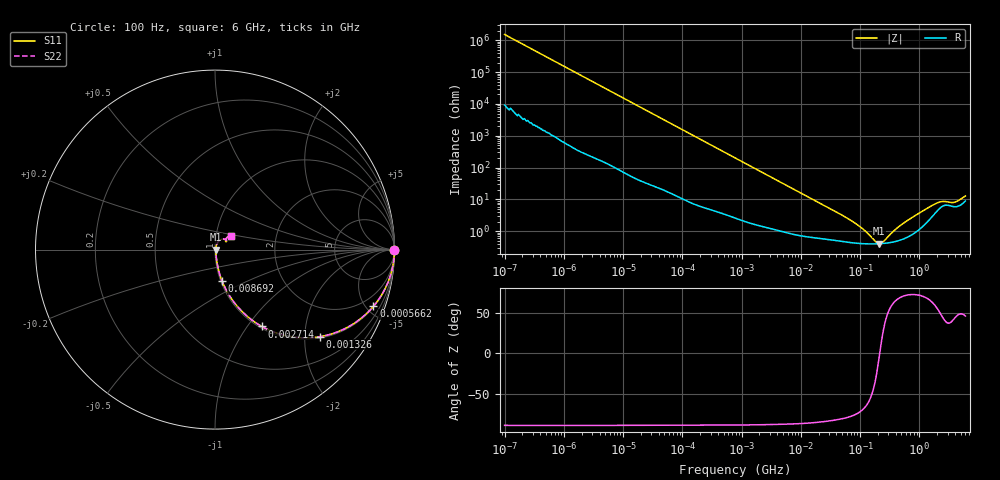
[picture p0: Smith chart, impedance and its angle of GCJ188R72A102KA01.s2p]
!Murata Part Number: GCJ188R72A102KA01
!These Parameters are Measured in Series Mode Connection
!Data Generated on Mar 13, 2026
!  o--ll--o
!Port1  Port2
!  o------o
!Operation Temp=25[degC], DC Bias Voltage=0[V]
!Freq. Start=100[Hz] Stop=6[GHz] 401[Steps]
# Hz S RI R 50
!Freq.(Hz) S11(Real) S11(Imag) S21(Real) S21(Imag) S12(Real) S12(Imag) S22(Real) S22(Imag)
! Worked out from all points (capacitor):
!   401 points, 100 Hz to 6 GHz, reference 50 ohm
!   read as one part in series: C = 1.04 nF near 109 Hz
!   lowest |Z| = 408 mohm at 208.8 MHz (marker M1)
!   series resonance near 214.7 MHz, so ESL is about 530 pH
!   S11 on the Smith chart (normalised r, x): 100 Hz: open; 566.2 kHz: 1.06, -5.55; 1.326 MHz: 1.04, -2.39; 2.714 MHz: 1.03, -1.17; 8.692 MHz: 1.02, -0.37; 6 GHz: 1.18, +0.19
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100  1 -6.54e-05  4e-07 6.54e-05  4e-07 6.54e-05  1 -6.54e-05
164  1 -0.000107  5e-07 0.000107  5e-07 0.000107  1 -0.000107
2008  1 -0.0013  6.8e-06 0.0013  6.8e-06 0.0013  1 -0.0013
40335  0.9992 -0.0259  0.000825 0.0259  0.000825 0.0259  0.9992 -0.0259
176758  0.9866 -0.1115  0.0134 0.1115  0.0134 0.1115  0.9866 -0.1115
566185  0.8824 -0.3164  0.1176 0.3164  0.1176 0.3164  0.8824 -0.3164
774597  0.8024 -0.3919  0.1976 0.3919  0.1976 0.3919  0.8024 -0.3919
1325623  0.586 -0.4849  0.414 0.4849  0.414 0.4849  0.586 -0.4849
2713602  0.2603 -0.4279  0.7397 0.4279  0.7397 0.4279  0.2603 -0.4279
4643984  0.1129 -0.3024  0.8871 0.3024  0.8871 0.3024  0.1129 -0.3024
8692127  0.0399 -0.1763  0.9601 0.1763  0.9601 0.1763  0.0399 -0.1763
1.555665e7  0.0168 -0.1013  0.9832 0.1013  0.9832 0.1013  0.0168 -0.1013
7.797396e7  0.00463 -0.0187  0.9954 0.0187  0.9954 0.0187  0.00463 -0.0187
1.825626e8  0.00401 -0.00257  0.996 0.00257  0.996 0.00257  0.00401 -0.00257
2.088084e8  0.00404 -0.00044  0.996 0.00044  0.996 0.00044  0.00404 -0.00044
2.388273e8  0.00411 0.00169  0.9959 -0.00169  0.9959 -0.00169  0.00411 0.00169
3.124326e8  0.00439 0.00608  0.9956 -0.00608  0.9956 -0.00608  0.00439 0.00608
5.847788e8  0.00641 0.0187  0.9936 -0.0187  0.9936 -0.0187  0.00641 0.0187
1.712697e9  0.0336 0.056  0.9664 -0.056  0.9664 -0.056  0.0336 0.056
2.34314e9  0.0577 0.0564  0.9423 -0.0564  0.9423 -0.0564  0.0577 0.0564
3.8344e9  0.0586 0.0487  0.9414 -0.0487  0.9414 -0.0487  0.0586 0.0487
6e9  0.0883 0.0782  0.9117 -0.0782  0.9117 -0.0782  0.0883 0.0782
